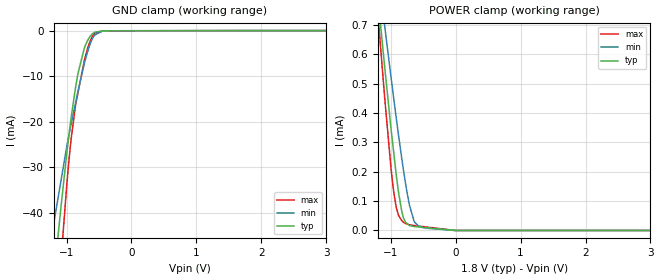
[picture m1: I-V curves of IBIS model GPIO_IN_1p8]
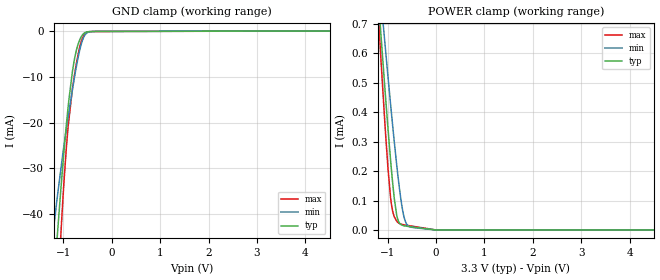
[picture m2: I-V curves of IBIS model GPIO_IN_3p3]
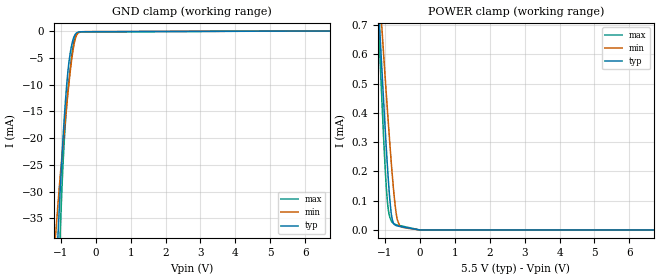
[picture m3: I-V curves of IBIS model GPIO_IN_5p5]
|Texas Instruments Incorporated
| Part#   Digital Voltage Range   Package-type   #pins
|  AMC7836   1.8V-5.5V   PQFP   64
[IBIS Ver]   4.1
[File name]   amc7836.ibs
[File Rev]   1.0
[Date]   06/26/2014
[Source]
| Texas Instruments Incorporated.
| 12500 TI Blvd
| Dallas, TX -75243
[Notes]   Revision History:
| Rev 1.0: 06/26/2014
| - Initial version of the model
| - Model generated from simulations in TISPICE
| - C_comp although listed in numerical order of value are
|   obtained from varying PVT conditions. For PVT conditions for
|   each specific value refer the buffer description under
|   respective [Model]. IBIS model user is responsible for using
|   appropriate C_comp to simulate for Signal Integrity.
| - Warnings regarding combined Non-monotonicity of various models have been
|   reviewd and considered minor and can be ignored.
| - Model names with a trailing _1p8 contains the model for
|   1.8V operation.Model names with a trailing _3p3 contains the model
|   for 3.3V operation.Model names with a trailing _5p5 contains the model
|   for 5.5V operation.
| - Please note GPIO model is broken into two models depending on its mode
|   of operation (output or input).
[Disclaimer]
| This model is designed as an aid for customers of Texas Instruments.
| TI and its licensors and suppliers make no warranties, either expressed
| or implied, with respect to this  model, including the warranties of
| merchantability or fitness for a particular purpose. The model is
| provided solely on an "as is" basis. The entire risk as to its quality
| and performance is with the customer.
[Copyright]
 (C) Copyright 2014 Texas Instruments Incorporated.All rights reserved.
|   Device
[Component]  amc7836
[Manufacturer]   TI
[Package]
| PQFP   64
|   typ   min   max
R_pkg   0.127   0.049   0.180
L_pkg   2.830nH   2.163nH   3.549nH
C_pkg   0.461pF   0.424pF   0.565pF
[Pin]  signal_name   model_name   R_pin   L_pin   C_pin
1   IOVDD   POWER   0.15239   3.13974nH   0.42606pF
2   RESETB   SDI   0.14796   3.04419nH   0.46725pF
3   SDO   SDO   0.143   2.95792nH   0.46112pF
4   SDI   SDI   0.14159   2.92462nH   0.45673pF
5   SCLK   SDI   0.1382   2.86378nH   0.45031pF
6   CS   SDI   0.13393   2.78603nH   0.44205pF
7   GPIO0/ALARMIN   GPIO   0.13165   2.74155nH   0.43418pF
8   GPIO1/ALARMOUT   GPIO   0.13019   2.71552nH   0.42524pF
9   GPIO2/ADCTRIG   GPIO   0.12924   2.70106nH   0.42431pF
10   GPIO3/DAV   GPIO   0.1291   2.70239nH   0.43179pF
11   GPIO4   GPIO   0.12979   2.72235nH   0.43732pF
12   GPIO5   GPIO   0.13131   2.75704nH   0.44477pF
13   GPIO6   GPIO   0.13446   2.81391nH   0.45417pF
14   GPIO7   GPIO   0.13795   2.87915nH   0.457pF
15   DAC_A0   NC   0.13627   2.86092nH   0.45521pF
16   DAC_A1   NC   0.15821   3.23194nH   0.43143pF
17   AVEE   GND   0.08469   2.88016nH   0.47657pF
18   DAC_A2   NC   0.15537   3.17054nH   0.48073pF
19   DAC_A3   NC   0.14591   3.01397nH   0.46944pF
20   AVCC_AB   POWER   0.05408   2.39897nH   0.55483pF
21   AGND1   GND   0.05469   2.42156nH   0.54737pF
22   DAC_B4   NC   0.15176   3.07398nH   0.46021pF
23   DAC_B5   NC   0.1445   2.94999nH   0.44909pF
24   AVSSB   GND   0.0757   2.48965nH   0.48105pF
25   DAC_B6   NC   0.14392   2.93664nH   0.43998pF
26   DAC_B7   NC   0.13889   2.86203nH   0.43907pF
27   ADC_15   NC   0.13909   2.87509nH   0.44528pF
28   ADC_14   NC   0.13319   2.79497nH   0.44897pF
29   ADC_13   NC   0.12937   2.744nH   0.45043pF
30   ADC_12   NC   0.12824   2.73744nH   0.45228pF
31   ADC_11   NC   0.1306   2.78203nH   0.45401pF
32   ADC_10   NC   0.15878   3.24917nH   0.43231pF
33   ADC_9   NC   0.16622   3.36593nH   0.44312pF
34   ADC_8   NC   0.15358   3.14086nH   0.47645pF
35   LV_ADC20   NC   0.14887   3.0586nH   0.46695pF
36   LV_ADC19   NC   0.14345   2.9618nH   0.45672pF
37   LV_ADC18   NC   0.14202   2.93016nH   0.45003pF
38   LV_ADC17   NC   0.1385   2.86288nH   0.44444pF
39   LV_ADC16   NC   0.13601   2.81327nH   0.44036pF
40   ADC_7   NC   0.1329   2.75958nH   0.433pF
41   ADC_6   NC   0.13296   2.75958nH   0.43347pF
42   ADC_5   NC   0.1353   2.79995nH   0.44282pF
43   ADC_4   NC   0.13979   2.87962nH   0.45189pF
44   ADC_3   NC   0.1465   2.99612nH   0.46345pF
45   ADC_2   NC   0.15531   3.14258nH   0.47875pF
46   ADC_1   NC   0.16646   3.3292nH   0.49392pF
47   ADC_0   NC   0.17986   3.54855nH   0.50046pF
48   AGND2   GND   0.06128   2.74647nH   0.51087pF
49   REF_CMP   NC   0.07658   2.54416nH   0.47195pF
50   AVDD   POWER   0.05483   2.36501nH   0.56532pF
51   DAC_C8   NC   0.14555   2.99746nH   0.47071pF
52   DAC_C9   NC   0.13851   2.87583nH   0.45762pF
53   AVSSC   GND   0.07198   2.39593nH   0.49304pF
54   DAC_C10   NC   0.13411   2.78691nH   0.44526pF
55   DAC_C11   NC   0.13128   2.7329nH   0.44006pF
56   AGND3   GND   0.0491   2.16292nH   0.51005pF
57   AVCC_CD   POWER   0.04996   2.1725nH   0.51584pF
58   DAC_D12   NC   0.13228   2.74849nH   0.44004pF
59   DAC_D13   NC   0.13054   2.73131nH   0.44037pF
60   AVSSD   GND   0.06871   2.30276nH   0.48762pF
61   DAC_D14   NC   0.13123   2.76243nH   0.45212pF
62   DAC_D15   NC   0.13448   2.82425nH   0.45538pF
63   DVDD   POWER   0.13565   2.85087nH   0.45818pF
64   DGND   GND   0.07511   2.51913nH   0.46159pF
|   Model Selectors
[Model Selector]  SDI
SDI_3p3   input buffer with 3.3V operation
SDI_1p8   input buffer with 1.8V operation
SDI_5p5   input buffer with 5.5V operation
[Model Selector]  SDO
SDO_3p3   output buffer with 3.3V operation
SDO_1p8   output buffer with 1.8V operation
SDO_5p5   output buffer with 5.5V operation
[Model Selector]  GPIO
GPIO_OUT_3p3   ouput mode with 3.3V operation
GPIO_OUT_1p8   ouput mode with 1.8V operation
GPIO_OUT_5p5   ouput mode with 5.5V operation
GPIO_IN_3p3   input mode with 3.3V operation
GPIO_IN_1p8   input mode with 1.8V operation
GPIO_IN_5p5   input mode with 5.5V operation
| Models and submodels in the file (12): GPIO_IN_1p8 (Input), GPIO_IN_3p3 (Input), GPIO_IN_5p5 (Input), GPIO_OUT_1p8 (Output), GPIO_OUT_3p3 (Output), GPIO_OUT_5p5 (Output), SDI_1p8 (Input), SDI_3p3 (Input), SDI_5p5 (Input), SDO_1p8 (Output), SDO_3p3 (Output), SDO_5p5 (Output)
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|   Model
[Model]   GPIO_IN_1p8
Model_type   Input
Vinl = 0.54
Vinh = 1.26
|   typ   min   max
C_comp   2.855pF   2.622pF   2.914pF
[Voltage Range]   1.8   1.79   1.81
[Temperature Range]   27   125   -40
[Power Clamp Reference]   1.8   1.79   1.81
[GND Clamp Reference]   0   0   0
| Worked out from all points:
|   GND clamp passes 1 mA (typ) near -0.62 V on its own axis
[GND Clamp]
|   Voltage   I(typ)   I(min)   I(max)
-1.8V     -152.4mA   -104.7mA   -207.8mA
-1.255V   -63.71mA   -47.78mA   -86.04mA
-1.195V   -54.51mA   -42.26mA   -73.13mA
-1.168V   -50.48mA   -39.98mA   -67.28mA
-1.093V   -39.73mA   -33.59mA   -51.85mA
-995.4mV  -26.89mA   -25.37mA   -33.77mA
-936.1mV  -19.9mA    -21.05mA   -24.76mA
-860.4mV  -12.45mA   -15.86mA   -16.27mA
-822.6mV  -9.362mA   -13.28mA   -13.56mA
-676.8mV  -2.207mA   -4.708mA   -3.996mA
-563.4mV  -354.6uA   -939uA     -593.4uA
3.6V      0A         0A         0A
[POWER Clamp]
|   Voltage   I(typ)   I(min)   I(max)
-1.8V     2.219mA    2.026mA    2.51mA
-1.17V    731.9uA    838.8uA    663.8uA
-1.152V   690.7uA    805.5uA    613.6uA
-1.093V   557.2uA    697.2uA    452.2uA
-1.068V   504.7uA    653uA      392.3uA
-952.2mV  262.9uA    447.8uA    128.8uA
-876.6mV  126uA      320.4uA    50.51uA
-828mV    63.72uA    242.8uA    33.09uA
-774mV    28.33uA    163.6uA    23.85uA
-639mV    13.56uA    31.19uA    16.8uA
-444.6mV  9.239uA    7.553uA    11.63uA
3.6V      0A         0A         0A
|   Model
[Model]   GPIO_IN_3p3
Model_type   Input
Vinl = 0.99
Vinh = 2.31
|   typ   min   max
C_comp   2.855pF   2.622pF   2.914pF
[Voltage Range]   3.3   3.29   3.31
[Temperature Range]   27   125   -40
[Power Clamp Reference]   3.3   3.29   3.31
[GND Clamp Reference]   0   0   0
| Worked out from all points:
|   GND clamp passes 1 mA (typ) near -0.62 V on its own axis
|   POWER clamp passes 1 mA (typ) near -1.29 V on its own axis
[GND Clamp]
|   Voltage   I(typ)   I(min)   I(max)
-3.3V     -417.9mA   -289mA     -553.3mA
-1.231V   -59.8mA    -45.81mA   -80.57mA
-1.191V   -53.9mA    -41.92mA   -72.16mA
-1.132V   -45.28mA   -36.61mA   -59.81mA
-1.053V   -34.32mA   -30.04mA   -44.13mA
-941.3mV  -20.52mA   -21.44mA   -25.5mA
-904.2mV  -16.57mA   -18.84mA   -20.85mA
-815.1mV  -8.835mA   -12.81mA   -12.55mA
-745.8mV  -4.737mA   -8.45mA    -7.85mA
-666.6mV  -1.965mA   -4.257mA   -3.564mA
-537.9mV  -251.4uA   -605.9uA   -378.3uA
6.6V      0A         0A         0A
[POWER Clamp]
|   Voltage   I(typ)   I(min)   I(max)
-3.3V     5.688mA    4.803mA    6.793mA
-1.171V   735.9uA    841.2uA    669.4uA
-1.132V   645.2uA    768.5uA    558.2uA
-1.063V   491uA      643.8uA    374.8uA
-993.3mV  343uA      519.2uA    208uA
-933.9mV  224.9uA    416.1uA    101.3uA
-815.1mV  51.97uA    223.1uA    30.18uA
-706.2mV  16.45uA    81.26uA    19.07uA
-646.8mV  13.78uA    35.08uA    17.01uA
-567.6mV  11.82uA    12.91uA    14.84uA
-3.3mV    30.97nA    10.63nA    56.2nA
6.6V      0A         0A         0A
|   Model
[Model]   GPIO_IN_5p5
Model_type   Input
Vinl = 1.65
Vinh = 3.85
|   typ   min   max
C_comp   2.855pF   2.622pF   2.914pF
[Voltage Range]   5.5   5.49   5.51
[Temperature Range]   27   125   -40
[Power Clamp Reference]   5.5   5.49   5.51
[GND Clamp Reference]   0   0   0
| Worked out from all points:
|   GND clamp passes 1 mA (typ) near -0.62 V on its own axis
|   POWER clamp passes 1 mA (typ) near -1.29 V on its own axis
[GND Clamp]
|   Voltage   I(typ)   I(min)   I(max)
-5.5V     -814.8mA   -579.3mA   -1.061A
-1.144V   -47.05mA   -37.71mA   -62.34mA
-1.078V   -37.78mA   -32.03mA   -49.05mA
-1.028V   -31.17mA   -28mA      -39.67mA
-1.012V   -29.05mA   -26.7mA    -36.71mA
-946mV    -21.08mA   -21.81mA   -26.2mA
-896.5mV  -15.85mA   -18.34mA   -20.03mA
-830.5mV  -10.04mA   -13.86mA   -13.79mA
-781mV    -6.626mA   -10.65mA   -10.19mA
-649mV    -1.593mA   -3.529mA   -2.88mA
-517mV    -228.9uA   -452.3uA   -313uA
11V       0A         0A         0A
[POWER Clamp]
|   Voltage   I(typ)   I(min)   I(max)
-5.5V     9.928mA    9.651mA    11.85mA
-1.226V   861.5uA    942.8uA    823.2uA
-1.161V   710uA      820.9uA    637.2uA
-1.144V   672.5uA    790.6uA    591.5uA
-1.111V   598.2uA    730.3uA    501.4uA
-1.045V   452.6uA    611uA      329.3uA
-929.5mV  216.6uA    408.6uA    95.49uA
-814mV    51.05uA    221.4uA    29.94uA
-682mV    15.05uA    58.94uA    18.11uA
-566.5mV  11.78uA    12.77uA    14.79uA
-5.5mV    55.86nA    23.26nA    96.36nA
11V       0A         0A         0A
